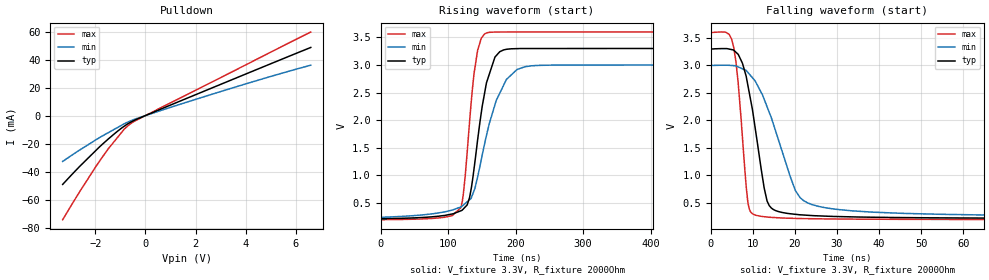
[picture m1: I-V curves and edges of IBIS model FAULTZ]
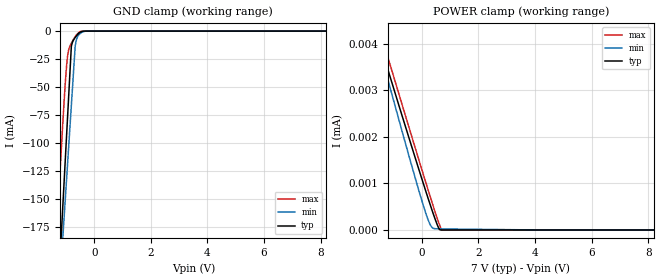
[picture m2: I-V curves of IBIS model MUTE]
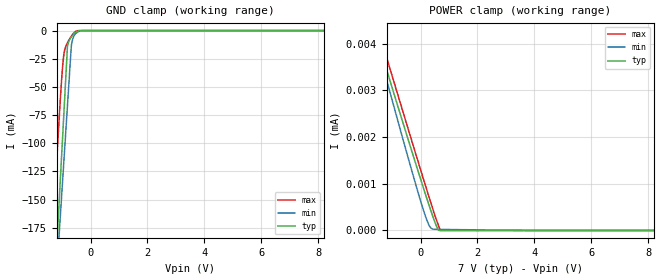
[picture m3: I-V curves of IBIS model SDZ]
|Texas Instruments Incorporated
| 20W MONO AUTOMOTIVE DIGITAL AMPLIFIER WITH DIAGNOSTICS
| Marketing part#   Digital Voltage Range   Package-type   #pins
| TAS5411   4.5V - 5.5V   WQFN   16
[IBIS Ver]   4.1
[File name]   tas5411_q1.ibs
[File Rev]   1.0
[Date]   03/26/2014
[Source]
| Texas Instruments Incorporated.
| 12500 TI Blvd
| Dallas, TX -75243
[Notes]   Revision History:
| Rev 1.0: 03/26/2014
| - Initial version of the model
| - Model generated from simulations in TISPICE
| - C_comp although listed in numerical order of value are
|   obtained from varying PVT conditions. For PVT conditions for
|   each specific value refer the buffer description under
|   respective [Model]. IBIS model user is responsible for using
|   appropriate C_comp to simulate for Signal Integrity.
| - Warnings regarding combined Non-monotonicity of various models have been
|   reviewd and considered minor and can be ignored.
[Disclaimer]
| This model is designed as an aid for customers of Texas Instruments.
| TI and its licensors and suppliers make no warranties, either expressed
| or implied, with respect to this  model, including the warranties of
| merchantability or fitness for a particular purpose. The model is
| provided solely on an "as is" basis. The entire risk as to its quality
| and performance is with the customer.
[Copyright]
 (C) Copyright 2014 Texas Instruments Incorporated.All rights reserved.
|   Device
[Component]   TAS5411
[Manufacturer]   TI
[Package]
| variable   typ   min   max
R_pkg   0.01   0.008   0.12
L_pkg   1.0nH   0.8nH   1.2nH
C_pkg   0.2pF   0.16pF   0.24pF
[Pin]  signal_name   model_name   R_pin   L_pin   C_pin
1   GND   GND   NA   NA   NA
2   STANDBYB   SDZ   NA   NA   NA
3   BYP   NC   NA   NA   NA
4   SDA   SDA   NA   NA   NA
5   SCL   SCL   NA   NA   NA
6   IN_P   NC   NA   NA   NA
7   IN_N   NC   NA   NA   NA
8   MUTE   MUTE   NA   NA   NA
9   GND   GND   NA   NA   NA
10   BSTN   NC   NA   NA   NA
11   OUTN   NC   NA   NA   NA
12   OUTP   NC   NA   NA   NA
13   BSTP   NC   NA   NA   NA
14   FAULTB   FAULTZ   NA   NA   NA
15   PVDD   POWER   NA   NA   NA
16   GND   GND   NA   NA   NA
| Models and submodels in the file (5): FAULTZ (Open_drain), MUTE (Input), SDZ (Input), SCL (Input), SDA (I/O_open_drain)
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|   Model
[Model]   FAULTZ
Model_type   Open_drain
Polarity   Non-Inverting
Vmeas = 1.65
Vref = 3.3
Cref = 1pF
Rref = 2000
|   typ   min   max
C_comp   1.124pF   1.094pF   1.139pF
[Voltage Range]   3.3   3   3.6
[Temperature Range]   27   125   -40
[Pullup Reference]   3.3   3   3.6
[Pulldown Reference]   0   0   0
[Power Clamp Reference]   3.3   3   3.6
[GND Clamp Reference]   0   0   0
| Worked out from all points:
|   slope of the pulldown table from 0 to 0.495 V, typ, clamps not added: 133 ohm
|   falling waveform, V_fixture 3.3V, R_fixture 2000Ohm: 20-80 % time 3.86ns typ, 7.41ns min, 2.15ns max; typ from 3.3 V to 0.211 V
|   rising waveform, V_fixture 3.3V, R_fixture 2000Ohm: 20-80 % time 21.8ns typ, 34.6ns min, 14.9ns max; typ from 0.211 V to 3.3 V
[Pulldown]
|   Voltage   I(typ)   I(min)   I(max)
-3.3V     -49.15mA   -32.73mA   -74.35mA
-2.637V   -36.55mA   -24.76mA   -54.77mA
-1.716V   -20.48mA   -14.53mA   -29.6mA
-1.478V   -16.67mA   -12.17mA   -23.66mA
-849.4mV  -7.666mA   -5.913mA   -9.822mA
-607.2mV  -4.904mA   -3.869mA   -6.03mA
-330mV    -2.501mA   -1.973mA   -3.015mA
2.927V    21.74mA    16.75mA    26.43mA
6.6V      48.68mA    36.02mA    59.74mA
[Ramp]
R_load = 2000
|   typ   min   max
dV/dt_r   1.85355/2.17879e-08   1.65622/3.46057e-08   2.04424/1.49217e-08
dV/dt_f   1.85355/3.85905e-09   1.65622/7.41174e-09   2.04424/2.1505e-09
[Falling Waveform]
V_fixture = 3.3V
V_fixture_min = 3V
V_fixture_max = 3.6V
R_fixture = 2000Ohm
C_fixture = 0F
|   Time   V(typ)   V(min)   V(max)
0s        3.3V       3V         3.6V
5.468ns   3.277V     2.997V     3.317V
7.511ns   3.041V     2.939V     1.689V
9.148ns   2.498V     2.843V     384.6mV
13.37ns   532.6mV    2.249V     241.2mV
16.99ns   323.6mV    1.426V     223.1mV
20.12ns   290.6mV    720.6mV    216.1mV
24.03ns   267.8mV    468.1mV    210.5mV
54.95ns   226mV      290.5mV    197.7mV
1us       210.7mV    239.6mV    192.9mV
[Rising Waveform]
V_fixture = 3.3V
V_fixture_min = 3V
V_fixture_max = 3.6V
R_fixture = 2000Ohm
C_fixture = 0F
|   Time   V(typ)   V(min)   V(max)
0s        210.7mV    239.6mV    192.9mV
119ns     354.2mV    423.7mV    411.1mV
125.3ns   421.9mV    485.7mV    976.8mV
131.9ns   597.7mV    554.8mV    1.981V
138.5ns   1.126V     721mV      2.852V
149.2ns   2.139V     1.285V     3.489V
157.9ns   2.719V     1.78V      3.587V
186.4ns   3.285V     2.738V     3.6V
223.2ns   3.3V       2.985V     3.6V
1us       3.3V       3V         3.6V
|   Model
[Model]   MUTE
Model_type   Input
Vinl = 0.9
Vinh = 2.31
|   typ   min   max
C_comp   1.258pF   1.202pF   1.424pF
[Voltage Range]   7   6.4   7.4
[Temperature Range]   27   125   -40
[Power Clamp Reference]   7   6.4   7.4
[GND Clamp Reference]   0   0   0
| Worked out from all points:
|   GND clamp passes 1 mA (typ) near -0.50 V on its own axis
|   POWER clamp passes 1 mA (typ) near -6.11 V on its own axis
[GND Clamp]
|   Voltage   I(typ)   I(min)   I(max)
-7V       -3.017A    -3.071A    -2.985A
-2.8V     -952.8mA   -991mA     -897.2mA
-1.26V    -224.4mA   -245.9mA   -146.9mA
-1.162V   -177.8mA   -202.1mA   -102mA
-1.099V   -148mA     -177.5mA   -74.55mA
-1.015V   -108.3mA   -144.7mA   -41.41mA
-952mV    -78.45mA   -120.1mA   -23.22mA
-815.1mV  -13.66mA   -66.58mA   -10.89mA
-679mV    -5.726mA   -13.41mA   -4.996mA
-616mV    -3.706mA   -6.376mA   -2.82mA
-490mV    -854.4uA   -1.874mA   -298.9uA
14V       0A         0A         0A
[POWER Clamp]
|   Voltage   I(typ)   I(min)   I(max)
-7V       1.573mA    1.876mA    1.501mA
-2.8V     6.617uA    6.819uA    6.955uA
-1.204V   3.453uA    3.234uA    3.715uA
-406mV    1.882uA    1.482uA    2.106uA
35mV      1.03uA     558.7nA    1.226uA
161mV     791.1nA    319.3nA    977.3nA
287mV     556.1nA    121.6nA    731.2nA
350mV     441.1nA    60.13nA    609.6nA
413mV     328.7nA    33.7nA     489.3nA
623mV     8.603nA    23.98nA    112.6nA
707mV     0A         23.14nA    520.6pA
14V       0A         0A         0A
|   Model
[Model]   SDZ
Model_type   Input
Vinl = 0.9
Vinh = 2.31
|   typ   min   max
C_comp   1.258pF   1.202pF   1.424pF
[Voltage Range]   7   6.4   7.4
[Temperature Range]   27   125   -40
[Power Clamp Reference]   7   6.4   7.4
[GND Clamp Reference]   0   0   0
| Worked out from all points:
|   GND clamp passes 1 mA (typ) near -0.50 V on its own axis
|   POWER clamp passes 1 mA (typ) near -6.11 V on its own axis
[GND Clamp]
|   Voltage   I(typ)   I(min)   I(max)
-7V       -3.017A    -3.071A    -2.985A
-2.8V     -952.8mA   -991mA     -897.2mA
-1.26V    -224.4mA   -245.9mA   -146.9mA
-1.162V   -177.8mA   -202.1mA   -102mA
-1.099V   -148mA     -177.5mA   -74.55mA
-1.015V   -108.3mA   -144.7mA   -41.41mA
-952mV    -78.45mA   -120.1mA   -23.22mA
-815.1mV  -13.66mA   -66.58mA   -10.89mA
-679mV    -5.726mA   -13.41mA   -4.996mA
-616mV    -3.706mA   -6.376mA   -2.82mA
-490mV    -854.4uA   -1.874mA   -298.9uA
14V       0A         0A         0A
[POWER Clamp]
|   Voltage   I(typ)   I(min)   I(max)
-7V       1.573mA    1.876mA    1.501mA
-2.8V     6.617uA    6.819uA    6.955uA
-1.204V   3.453uA    3.234uA    3.715uA
-406mV    1.882uA    1.482uA    2.106uA
35mV      1.03uA     558.6nA    1.226uA
161mV     791.1nA    319.3nA    977.3nA
287mV     556.1nA    121.5nA    731.2nA
350mV     441.1nA    59.94nA    609.6nA
413mV     328.7nA    33.37nA    489.3nA
623mV     8.499nA    23.61nA    112.6nA
707mV     0A         22.77nA    388.9pA
14V       0A         0A         0A
